FUNCTION FC 118 : VOID
TITLE =COPY OF THE HANDLING PROGRAM > WORKING AREA
AUTHOR : Esposito
FAMILY : EGAL_srl
NAME : CO_DB_DB
VERSION : 0.1

BEGIN
NETWORK
TITLE =HANDLING PROGRAM > WORKING AREA

      U     M     47.3;
      U     E     21.0;
      SPB   HAND;
      SPA   NOTH;

HAND: L     DB16.DBD  158;
      T     DB15.DBD  158;

      L     DB16.DBD  134;
      T     DB15.DBD  134;

      L     DB16.DBD  126;
      T     DB15.DBD  126;

      L     DB16.DBW  276;
      T     DB15.DBW  276;

      L     DB16.DBW   22;
      T     DB15.DBW   22;

      L     DB16.DBW   24;
      T     DB15.DBW   24;

      L     DB16.DBW   26;
      T     DB15.DBW   26;

      L     DB16.DBW   28;
      T     DB15.DBW   28;

      L     DB16.DBW   30;
      T     DB15.DBW   30;

      L     DB16.DBW   32;
      T     DB15.DBW   32;

      L     DB16.DBW   34;
      T     DB15.DBW   34;

      L     DB16.DBW   36;
      T     DB15.DBW   36;

      L     DB16.DBW  208;
      T     DB15.DBW  208;

      L     DB16.DBW  210;
      T     DB15.DBW  210;

      L     DB16.DBW   50;
      T     DB15.DBW   50;

      L     DB16.DBW   52;
      T     DB15.DBW   52;

      L     DB16.DBW  212;
      T     DB15.DBW  212;

      L     DB16.DBW  214;
      T     DB15.DBW  214;

      L     DB16.DBW  216;
      T     DB15.DBW  216;

      L     DB16.DBW  218;
      T     DB15.DBW  218;

      L     DB16.DBW  220;
      T     DB15.DBW  220;

      L     DB16.DBW  222;
      T     DB15.DBW  222;

      L     DB16.DBW  224;
      T     DB15.DBW  224;

      L     DB16.DBW  226;
      T     DB16.DBW  226;

      L     DB16.DBW  194;
      T     DB15.DBW  194;

      L     DB16.DBW  196;
      T     DB15.DBW  196;

      L     DB16.DBW  198;
      T     DB16.DBW  198;

NOTH: NOP   0;






END_FUNCTION

